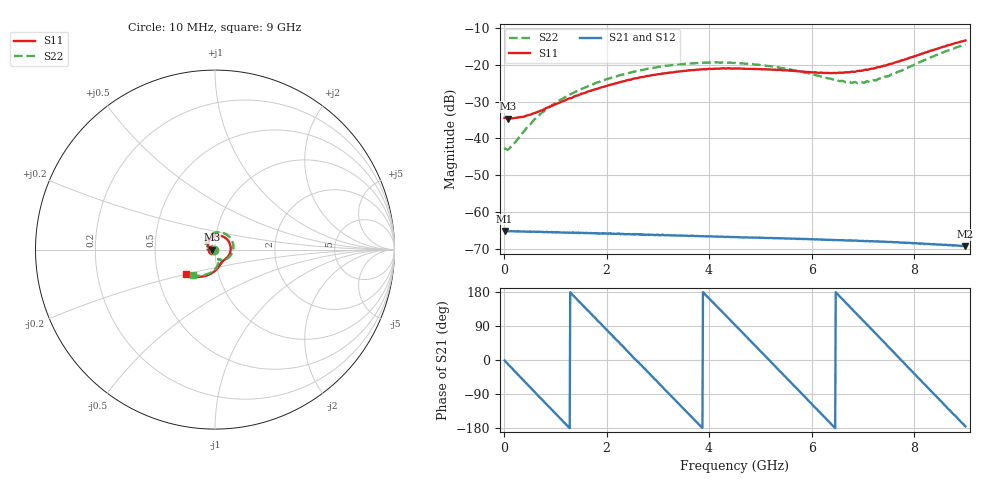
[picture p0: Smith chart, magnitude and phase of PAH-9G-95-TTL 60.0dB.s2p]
! MTS Systemtechnik GmbH
! S-Parameters
! Model: PAH-9G/95-TTL
! Attenuation Step: 50.0dB
#  HZ  S  DB  R  50.00
! Rohde & Schwarz Vector Network Analyzer
! Rohde-Schwarz,ZNB20-2Port,1334333062101652,3.45
! Created: UTC 1/26/2024, 7:22:43 AM
! freq[Hz]  db:S11  ang:S11  db:S21  ang:S21  db:S12  ang:S12  db:S22  ang:S22
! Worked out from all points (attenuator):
!   900 points, 10 MHz to 9 GHz, reference 50 ohm
!   highest |S21| = -65.14 dB at 10 MHz (marker M1); lowest = -69.3 dB at 9 GHz (marker M2)
!   lowest |S11| = -34.6 dB at 80 MHz (marker M3), VSWR 1.04, Z = 48.2 - j0.0383 ohm
!   |S11| at or under -10 dB: start of sweep to end of sweep
!   |S22| runs from -43.1 to -14.5 dB; largest |S21 - S12| = 2e-05
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1e7  -34.44 -173.5  -65.14 -1.3  -65.16 -1.4  -42.57 -162.0
8e7  -34.61 -178.8  -65.23 -11.8  -65.24 -11.6  -43.04 -167.0
2.3e8  -34.42 -178.4  -65.32 -32.7  -65.29 -33.2  -40.85 -149.9
3.7e8  -34.15 -177.8  -65.30 -52.8  -65.33 -52.8  -38.38 -145.3
4.7e8  -33.70 -177.5  -65.35 -66.8  -65.42 -66.7  -36.61 -145.1
7.3e8  -32.44 179.7  -65.40 -103.0  -65.46 -103.0  -33.11 -152.3
1.08e9  -30.31 171.7  -65.53 -151.9  -65.57 -151.6  -29.67 -168.0
1.51e9  -27.89 157.8  -65.67 148.0  -65.72 148.3  -26.58 169.5
2.14e9  -25.17 131.0  -65.96 59.8  -65.96 60.5  -23.31 136.6
2.53e9  -23.78 113.6  -66.02 5.5  -66.06 6.7  -21.89 116.3
3.01e9  -22.56 91.9  -66.21 -60.3  -66.31 -60.3  -20.58 91.6
3.78e9  -21.33 55.8  -66.56 -167.0  -66.60 -166.7  -19.52 52.9
4.51e9  -21.02 22.2  -66.85 91.9  -66.86 92.0  -19.49 16.8
5.2e9  -21.30 -8.9  -67.08 -4.3  -67.13 -3.5  -20.38 -16.6
6.01e9  -22.08 -39.9  -67.36 -117.3  -67.45 -115.9  -22.55 -50.9
6.54e9  -22.14 -55.9  -67.67 168.5  -67.72 170.5  -24.44 -65.2
6.9e9  -21.67 -64.8  -67.83 118.3  -67.88 119.8  -24.97 -68.7
7.14e9  -21.12 -70.2  -68.02 85.5  -67.97 86.3  -24.62 -69.1
7.51e9  -19.84 -80.0  -68.15 33.3  -68.22 34.2  -23.06 -72.2
8.24e9  -16.60 -106.1  -68.72 -69.3  -68.70 -67.3  -18.49 -94.9
8.67e9  -14.66 -124.4  -69.01 -129.6  -69.02 -127.1  -16.08 -114.5
9e9  -13.39 -139.9  -69.30 -175.2  -69.35 -173.7  -14.51 -130.6
